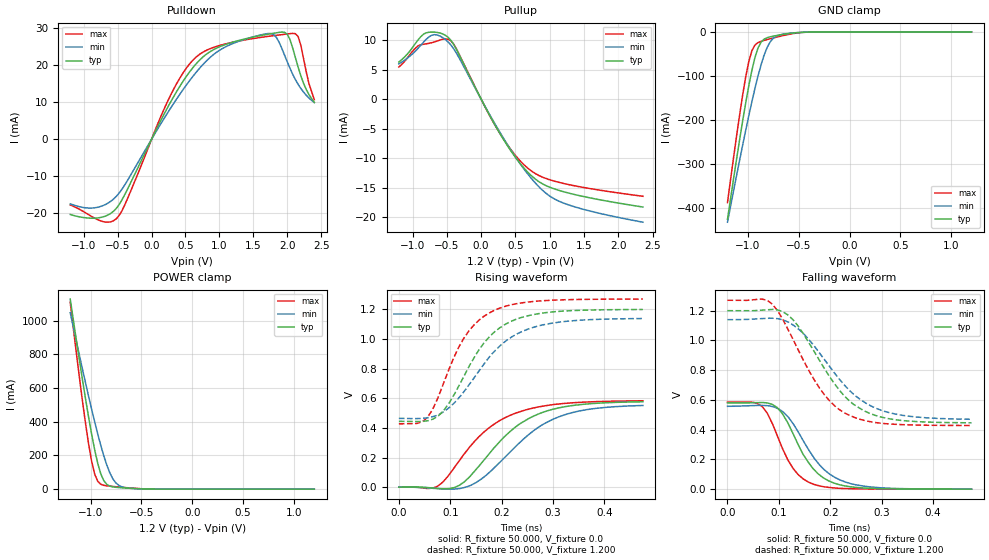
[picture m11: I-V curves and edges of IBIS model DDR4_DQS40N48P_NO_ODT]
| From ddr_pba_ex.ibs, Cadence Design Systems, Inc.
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|   Model DDR4_DQS40N48P_NO_ODT
[Model]   DDR4_DQS40N48P_NO_ODT
Model_type I/O
Polarity   Non-Inverting
Enable   Active-High
Vinl =  0.823V
Vinh =  0.887V
C_comp   1.707pF   1.713pF   1.723pF
C_comp_pullup   0.527pF   0.579pF   0.519pF
C_comp_pulldown   1.180pF   1.134pF   1.204pF
[Model Spec]
Vinh   0.887V   NA   NA
Vinl   0.823V   NA   NA
Vmeas   0.840V   NA   NA
[Temperature Range]   27.000   0.125k   -40.000
[Voltage Range]   1.200V   1.140V   1.270V
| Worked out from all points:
|   slope of the pulldown table from 0 to 0.18 V, typ, clamps not added: 27.2 ohm
|   slope of the pullup table from 0 to 0.18 V, typ, clamps not added: 45.9 ohm
|   GND clamp passes 1 mA (typ) near -0.50 V on its own axis
|   POWER clamp passes 1 mA (typ) near -0.46 V on its own axis
|   rising waveform, R_fixture 50.000, V_fixture 0.0: 20-80 % time 103ps typ, 110ps min, 100ps max; typ from 0 V to 0.577 V
|   rising waveform, R_fixture 50.000, V_fixture 1.200: 20-80 % time 83.7ps typ, 99.1ps min, 72.9ps max; typ from 0.445 V to 1.2 V
|   falling waveform, R_fixture 50.000, V_fixture 0.0: 20-80 % time 58.1ps typ, 68.4ps min, 49.4ps max; typ from 0.579 V to 0 V
|   falling waveform, R_fixture 50.000, V_fixture 1.200: 20-80 % time 89.4ps typ, 99.9ps min, 84.3ps max; typ from 1.2 V to 0.446 V
[Pulldown]
|Voltage   I(typ)   I(min)   I(max)
-1.2V     -20.33mA   -17.47mA   -17.73mA
-840mV    -21.33mA   -18.52mA   -21.33mA
-520mV    -18.67mA   -15.43mA   -21.47mA
400mV     13.8mA     11.7mA     16mA
640mV     20.01mA    17.69mA    21.92mA
960mV     24.62mA    23.51mA    25.09mA
1.76V     28.51mA    28.56mA    27.88mA
1.84V     28.75mA    27.53mA    28.07mA
2V        28.39mA    20.97mA    28.43mA
2.12V     22.12mA    16.15mA    28.52mA
2.2V      17.21mA    13.75mA    25.48mA
2.4V      9.967mA    9.905mA    10.69mA
[Pullup]
|Voltage   I(typ)   I(min)   I(max)
-1.2V     6.276mA    5.968mA    5.424mA
-960mV    9.396mA    8.108mA    8.597mA
-840mV    10.98mA    9.634mA    9.283mA
-720mV    11.33mA    10.8mA     9.54mA
-560mV    11.02mA    10.4mA     10.13mA
-400mV    9.244mA    8.51mA     9.292mA
280mV     -5.933mA   -5.721mA   -5.889mA
520mV     -10.14mA   -10.1mA    -9.786mA
760mV     -13.22mA   -13.77mA   -12.36mA
960mV     -14.69mA   -16.04mA   -13.47mA
1.2V      -15.64mA   -17.56mA   -14.24mA
2.36V     -18.24mA   -20.8mA    -16.42mA
[GND_clamp]
|Voltage   I(typ)   I(min)   I(max)
-1.2V     -426.2mA   -432.8mA   -388.3mA
-1.08V    -244.1mA   -290.9mA   -187.6mA
-1.02V    -160.2mA   -222.9mA   -101.2mA
-990mV    -121.8mA   -190.1mA   -66.76mA
-960mV    -87.12mA   -158.5mA   -42.47mA
-900mV    -36.37mA   -100.2mA   -23.99mA
-840mV    -16.17mA   -52.6mA    -18.98mA
-810mV    -12.75mA   -34.94mA   -17.06mA
-750mV    -9.219mA   -14.09mA   -13.42mA
-600mV    -3.476mA   -2.979mA   -5.372mA
-390mV    -77.95uA   -145.6uA   -88.64uA
1.2V      1.562nA    185.8nA    255.1pA
[POWER_clamp]
|Voltage   I(typ)   I(min)   I(max)
-1.2V     1.129A     1.047A     1.109A
-1.08V    651.1mA    713.3mA    524.8mA
-1.02V    430.1mA    553.1mA    270.8mA
-990mV    328mA      475.7mA    167mA
-960mV    234.7mA    400.6mA    90.32mA
-930mV    154.2mA    328.7mA    47.17mA
-900mV    91.53mA    260.8mA    29.3mA
-840mV    28.2mA     142.5mA    19.67mA
-780mV    13.3mA     60.49mA    15.94mA
-720mV    9.309mA    21.57mA    12.7mA
-660mV    6.902mA    8.818mA    9.642mA
1.2V      -4.11nA    -153.5nA   -871.8pA
[Ramp]
| variable   typ   min   max
dV/dt_r 0.348/0.105n   0.332/0.116n   0.351/0.105n
dV/dt_f 0.453/94.978p   0.403/0.104n   0.505/85.945p
R_load = 50.000
| The next line is not an IBIS keyword
| [Initial Delay]   0.300ns   0.500ns   0.200ns
[Rising Waveform]
R_fixture= 50.000
V_fixture= 0.0
V_fixture_min= 0.0
V_fixture_max= 0.0
|time   V(typ)   V(min)   V(max)
0s        369.8uV    1.134mV    452.1uV
75ps      -8.28mV    -9.428mV   5.873mV
95ps      -10.37mV   -12.66mV   71.55mV
117ps     11.27mV    -9.493mV   176.4mV
166ps     185.2mV    69.85mV    373.8mV
226ps     403.9mV    270.7mV    498.6mV
269ps     490.4mV    398.6mV    540mV
319ps     540.9mV    484.9mV    564.4mV
379ps     565.3mV    530.3mV    577.1mV
475ps     576.6mV    551.6mV    583.4mV
[Rising Waveform]
R_fixture= 50.000
V_fixture= 1.200
V_fixture_min= 1.140
V_fixture_max= 1.270
|time   V(typ)   V(min)   V(max)
0s        444.8mV    464.8mV    427.9mV
46ps      444.1mV    465.1mV    442.7mV
65ps      458.2mV    475.2mV    520.2mV
78ps      485.5mV    490.2mV    620.4mV
126ps     744.9mV    642.2mV    1.003V
156ps     927.7mV    785.3mV    1.127V
185ps     1.045V     913.5mV    1.192V
229ps     1.134V     1.033V     1.238V
279ps     1.175V     1.095V     1.258V
475ps     1.199V     1.138V     1.27V
[Falling Waveform]
R_fixture= 50.000
V_fixture= 0.0
V_fixture_min= 0.0
V_fixture_max= 0.0
|time   V(typ)   V(min)   V(max)
0s        579.3mV    557mV      585.2mV
67ps      582.9mV    563.3mV    557.3mV
77ps      580mV      561.6mV    513.5mV
96ps      550.6mV    545.5mV    367.1mV
127ps     378mV      444.2mV    142.4mV
146ps     240.5mV    334mV      72.52mV
167ps     136.9mV    216.8mV    33.63mV
199ps     52.77mV    100.9mV    10.92mV
248ps     12.5mV     30.38mV    2.348mV
475ps     173.6uV    242.9uV    61.55uV
[Falling Waveform]
R_fixture= 50.000
V_fixture= 1.200
V_fixture_min= 1.140
V_fixture_max= 1.270
|time   V(typ)   V(min)   V(max)
0s        1.2V       1.139V     1.27V
77ps      1.207V     1.149V     1.27V
97ps      1.206V     1.147V     1.202V
116ps     1.176V     1.127V     1.087V
137ps     1.099V     1.08V      940mV
177ps     876.8mV    925.5mV    690.1mV
227ps     629.1mV    702.1mV    513.6mV
265ps     528.4mV    588mV      463mV
309ps     477mV      519.6mV    440mV
475ps     446.1mV    469.7mV    428.1mV
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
